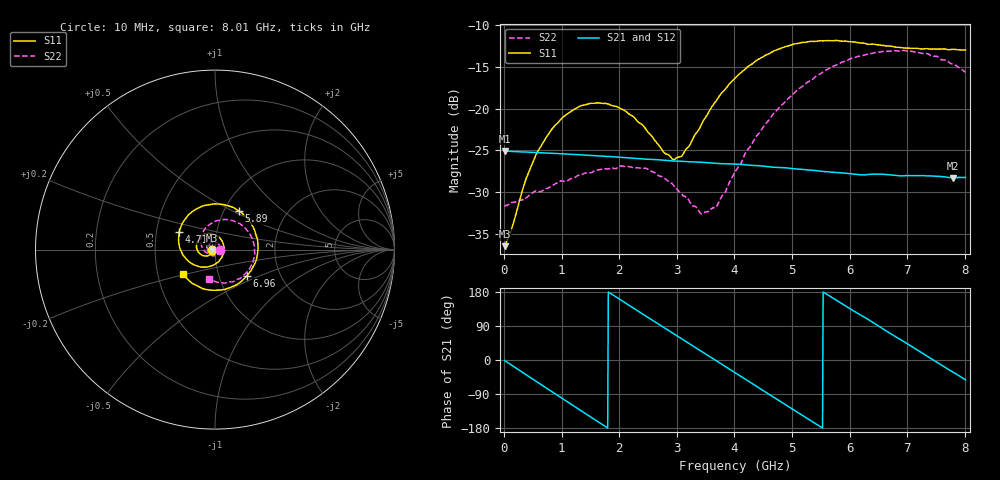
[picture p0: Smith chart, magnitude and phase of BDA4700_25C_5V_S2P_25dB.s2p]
!Agilent Technologies,E5071B,MY42404982,A.09.10
!Date: Mon Oct 20 13:39:03 2025
!Data & Calibration Information:
!Freq	S11:SOLT2(ON)	S21:SOLT2(ON)	S12:SOLT2(ON)	S22:SOLT2(ON)
# Hz S RI R 50
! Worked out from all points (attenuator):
!   801 points, 10 MHz to 8.01 GHz, reference 50 ohm
!   highest |S21| = -25.08 dB at 10 MHz (marker M1); lowest = -28.3 dB at 7.8 GHz (marker M2)
!   lowest |S11| = -36.5 dB at 10 MHz (marker M3), VSWR 1.03, Z = 48.5 - j0.129 ohm
!   |S11| at or under -10 dB: start of sweep to end of sweep
!   |S22| runs from -32.6 to -13.0 dB; largest |S21 - S12| = 0.00045
!   S11 on the Smith chart (normalised r, x): 10 MHz: 0.97, -0.00; 4.71 GHz: 0.66, +0.14; 5.89 GHz: 1.17, +0.54; 6.96 GHz: 1.36, -0.42; 8.01 GHz: 0.67, -0.19
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1e7  -0.0149 -0.00132  0.0557 -0.00118  0.0557 -0.00128  0.0262 -0.000795
1.2e8  -0.016 -0.00902  0.054 -0.0119  0.054 -0.0119  0.0266 -0.00579
3.8e8  -0.0265 -0.0266  0.0429 -0.0342  0.0428 -0.0342  0.0213 -0.0197
5.9e8  -0.0431 -0.0355  0.0276 -0.047  0.0276 -0.047  0.0134 -0.029
9.9e8  -0.0829 -0.0243  -0.00874 -0.0529  -0.00877 -0.0529  -0.0141 -0.0339
1.35e9  -0.1034 0.014  -0.0373 -0.0373  -0.0374 -0.0373  -0.0362 -0.0178
2.07e9  -0.0425 0.0886  -0.0458 0.0222  -0.0458 0.0222  -0.0304 0.0333
2.68e9  0.0409 0.0447  -0.00422 0.0491  -0.00418 0.0491  0.013 0.0375
2.93e9  0.0496 0.00147  0.016 0.0459  0.016 0.0458  0.0249 0.0247
3.06e9  0.0461 -0.0226  0.0255 0.0411  0.0253 0.0412  0.0276 0.0146
3.44e9  -0.002 -0.0821  0.0443 0.0176  0.0443 0.0176  0.0186 -0.0142
3.69e9  -0.0553 -0.0974  0.0469 -0.00192  0.047 -0.00208  0.000472 -0.0258
4.01e9  -0.1306 -0.0771  0.0389 -0.0255  0.0389 -0.0254  -0.0324 -0.0259
4.71e9  -0.1996 0.1003  -0.00841 -0.0437  -0.00826 -0.0437  -0.08 0.0526
5.35e9  -0.0555 0.2464  -0.0407 -0.0129  -0.0407 -0.013  -0.0156 0.1482
5.89e9  0.1335 0.2152  -0.0343 0.0227  -0.0343 0.0226  0.1049 0.159
6.26e9  0.2201 0.1094  -0.0155 0.0369  -0.0151 0.037  0.1815 0.1038
6.68e9  0.2315 -0.0506  0.012 0.0383  0.0121 0.0383  0.2203 0.000202
6.96e9  0.179 -0.1452  0.0272 0.0288  0.0272 0.0287  0.2089 -0.0759
7.37e9  0.0413 -0.2243  0.0391 0.00544  0.0392 0.00537  0.1369 -0.1622
7.8e9  -0.1225 -0.1903  0.0324 -0.0206  0.0325 -0.0207  0.0198 -0.1829
8.01e9  -0.1798 -0.1347  0.0237 -0.0306  0.0237 -0.0306  -0.0309 -0.162
